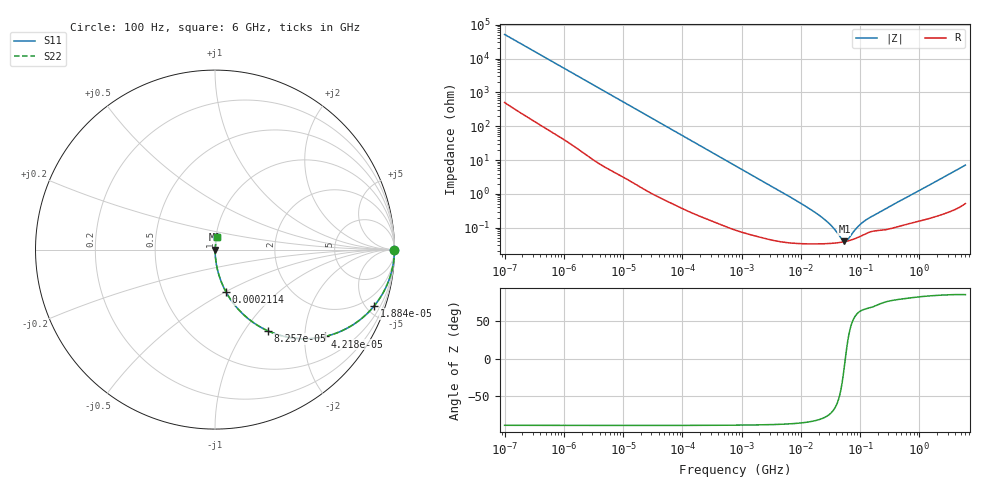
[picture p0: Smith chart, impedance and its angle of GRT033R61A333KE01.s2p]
!Murata Part Number: GRT033R61A333KE01
!These Parameters are Measured in Series Mode Connection
!Data Generated on Jun 19, 2026
!  o--ll--o
!Port1  Port2
!  o------o
!Operation Temp=25[degC], DC Bias Voltage=0[V]
!Freq. Start=100[Hz] Stop=6[GHz] 401[Steps]
# Hz S RI R 50
!Freq.(Hz) S11(Real) S11(Imag) S21(Real) S21(Imag) S12(Real) S12(Imag) S22(Real) S22(Imag)
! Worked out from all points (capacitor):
!   401 points, 100 Hz to 6 GHz, reference 50 ohm
!   read as one part in series: C = 30.7 nF near 109 Hz
!   lowest |Z| = 39.4 mohm at 54.5 MHz (marker M1)
!   series resonance near 56.44 MHz, so ESL is about 260 pH
!   S11 on the Smith chart (normalised r, x): 100 Hz: open; 18.84 kHz: 1.03, -5.63; 42.18 kHz: 1.02, -2.52; 82.57 kHz: 1.01, -1.29; 211.4 kHz: 1.00, -0.51; 6 GHz: 1.01, +0.14
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100  1 -0.00193  2.26e-05 0.00193  2.26e-05 0.00193  1 -0.00193
2008  0.9983 -0.0381  0.00171 0.0381  0.00171 0.0381  0.9983 -0.0381
7036  0.9818 -0.1307  0.0182 0.1307  0.0182 0.1307  0.9818 -0.1307
18841  0.8864 -0.3144  0.1136 0.3144  0.1136 0.3144  0.8864 -0.3144
26957  0.7935 -0.4019  0.2065 0.4019  0.2065 0.4019  0.7935 -0.4019
40335  0.6336 -0.4788  0.3664 0.4788  0.3664 0.4788  0.6336 -0.4788
42182  0.6128 -0.4841  0.3872 0.4841  0.3872 0.4841  0.6128 -0.4841
57709  0.4597 -0.4952  0.5403 0.4952  0.5403 0.4952  0.4597 -0.4952
82567  0.2952 -0.4528  0.7048 0.4528  0.7048 0.4528  0.2952 -0.4528
129199  0.1476 -0.3511  0.8524 0.3511  0.8524 0.3511  0.1476 -0.3511
211427  0.0618 -0.2368  0.9382 0.2368  0.9382 0.2368  0.0618 -0.2368
774597  0.00565 -0.069  0.9944 0.069  0.9944 0.069  0.00565 -0.069
1.555665e7  0.000343 -0.00323  0.9997 0.00323  0.9997 0.00323  0.000343 -0.00323
2.911731e7  0.000343 -0.00137  0.9997 0.00137  0.9997 0.00137  0.000343 -0.00137
3.64232e7  0.000352 -0.000869  0.9996 0.000869  0.9996 0.000869  0.000352 -0.000869
4.983056e7  0.000377 -0.000239  0.9996 0.000239  0.9996 0.000239  0.000377 -0.000239
5.449875e7  0.000388 -6.66e-05  0.9996 6.66e-05  0.9996 6.66e-05  0.000388 -6.66e-05
6.233367e7  0.000409 0.00019  0.9996 -0.00019  0.9996 -0.00019  0.000409 0.00019
8.918374e7  0.000506 0.000882  0.9995 -0.000882  0.9995 -0.000882  0.000506 0.000882
1.166697e8  0.000633 0.00142  0.9994 -0.00142  0.9994 -0.00142  0.000633 0.00142
3.124326e8  0.00094 0.00409  0.9991 -0.00409  0.9991 -0.00409  0.00094 0.00409
6e9  0.0101 0.0699  0.9899 -0.0699  0.9899 -0.0699  0.0101 0.0699
